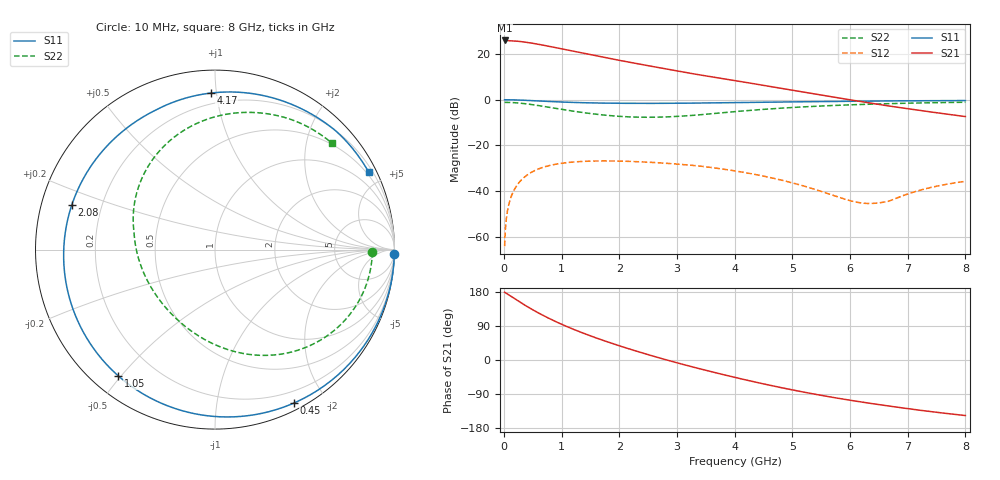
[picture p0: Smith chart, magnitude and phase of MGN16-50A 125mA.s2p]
! Port[1] = GATE
! Port[2] = DRAIN
! [Type]  S-parameter s2p file touchstone ver. 1.0
! [Object]  MGN16-50A
! [Bias]  125 mA
! [Version]  1.0
! [Date]  Thu May 28 10:54:03 2026
! [Source]  This file was created in JSC "ICC Milandr".
! [Disclaimer] Property of JSC "ICC Milandr". Unauthorized reproduction and/or distribution is strictly prohibited.
!  The file and the data are provided "AS IS" and with all faults and disclaim all warranties, express and implied, including
!  without limitation any implied warranties of merchantability, fitness for a particular purpose.
!  JSC "ICC Milandr" assumes no liability for:
!  1) the accuracy of the data provided;
!  2) the proper functioning of this data;
!  3) infringement of patents, copyrights or intellectual property rights resulting from the use of this data.
!  JSC "ICC Milandr" reserves the right to make changes to the products and the data without prior notice.
!  Please, be aware that your receipt and use of the file provided shall serve as acceptance of these terms and conditions.
!  If you do not accept these terms, you should return or destroy this file and any other accompanying information immediately.
# hz S ma R 12.5
! 2 Port Network Data from SP1.SP block
! freq  magS11  angS11  magS21  angS21  magS12  angS12  magS22  angS22
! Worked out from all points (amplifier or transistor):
!   800 points, 10 MHz to 8 GHz, reference 12.5 ohm
!   highest |S21| = 25.9 dB at 10 MHz (marker M1)
!   |S21| within 3 dB of that: start of sweep to 867.2 MHz
!   unconditionally stable (mu >= 1): 4.281 GHz to end of sweep
!   at 1.34 GHz: K = 0.19, MSG = 23.8 dB, |S12| = -27.0 dB
!   at 4.01 GHz: K = 0.86, MSG = 19.8 dB, |S12| = -31.2 dB
!   at 8 GHz: K = 1.17, MAG = 11.7 dB, |S12| = -35.7 dB
!   S11 on the Smith chart (normalised r, x): 10 MHz: 2, -79; 450 MHz: 0.07, -1.63; 1.05 GHz: 0.08, -0.49; 2.08 GHz: 0.09, +0.15; 4.17 GHz: 0.13, +0.96; 8 GHz: 0.39, +4.19
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1e7  0.9993 -1.4  19.81 178.9  0.0006263 82.2  0.8765 -0.8
4e7  0.999 -5.9  19.75 175.9  0.002478 84.4  0.876 -3.4
1e8  0.997 -14.7  19.62 169.9  0.006152 79.6  0.8719 -8.5
2e8  0.9904 -29.1  19.23 160.0  0.01206 70.5  0.8579 -16.8
3.3e8  0.9768 -47.1  18.45 147.6  0.01912 58.7  0.8286 -27.2
4.5e8  0.9613 -62.8  17.55 136.7  0.02481 48.4  0.7938 -36.2
5.8e8  0.9433 -78.8  16.47 125.5  0.03002 37.9  0.7517 -45.4
7.1e8  0.9255 -93.6  15.35 115.1  0.03426 28.0  0.7081 -54.0
8.6e8  0.9066 -109.4  14.08 103.9  0.03808 17.5  0.6593 -63.3
1.05e9  0.8862 -127.4  12.59 90.9  0.04154 5.2  0.6026 -74.2
1.2e9  0.8731 -140.2  11.51 81.3  0.04341 -3.8  0.563 -82.4
1.35e9  0.8623 -151.9  10.53 72.2  0.04467 -12.2  0.5285 -90.3
1.68e9  0.8458 -174.6  8.7 53.8  0.04584 -29.4  0.4696 -107.2
2.08e9  0.8357 162.6  6.961 33.6  0.04523 -48.2  0.4273 -127.8
2.38e9  0.8331 148.2  5.921 19.5  0.04379 -61.3  0.4145 -143.6
2.68e9  0.8339 135.6  5.052 6.1  0.04178 -73.8  0.4162 -159.3
3.27e9  0.8431 115.1  3.715 -18.3  0.03666 -97.0  0.4546 171.1
4.01e9  0.8672 95.4  2.614 -46.1  0.02768 -117.0  0.5506 140.7
4.17e9  0.8724 91.6  2.422 -51.8  0.02559 -120.7  0.5724 134.8
5.34e9  0.9078 67.0  1.369 -88.8  0.01145 -135.3  0.7138 97.3
6.67e9  0.9431 44.8  0.731 -121.3  0.006033 -74.4  0.8214 65.7
8e9  0.9594 26.6  0.4284 -146.6  0.01644 -61.2  0.8812 42.3
